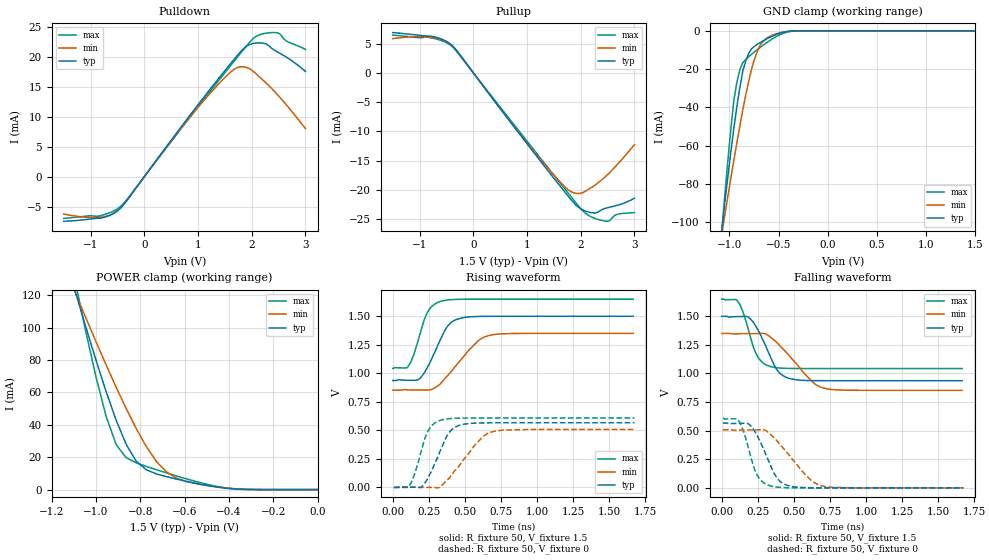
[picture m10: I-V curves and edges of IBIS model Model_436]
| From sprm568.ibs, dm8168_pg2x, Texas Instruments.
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| Model based on original model for BSHTLTCSCDDVGPBFZ
|   Sub model SLOW_5MA_10PER_N_1P5
[model]   Model_436
|[Description]  [1.5V-3-STATE-X-SLOW:5MA, IND, 10%]
|   Slow slew rate (SR[1:0] = "01"), 1.60 * RExt = 0.625 * Iout
|   (I[2:0] = "000"), 5mA nominal with Rext = 50R, ,Industrial
|   temperature range (-40C to 125C, 25C nominal),10% power supply
|   tolerance
|[Input Load]
|[Output Drive] SLOW:5MA
|Voltage   1.5V
|Mode   3-STATE
Model_type   3-state
Polarity   Non-Inverting
Enable   Active-Low
Cref =  15.0000pF
Rref =  100.0000M
Vref =  0V
Vmeas =  0.75
C_comp   1.5249p   1.4275p   1.6205p
[Model Spec]
[Temperature Range]   25   125   -40
[Voltage Range]   1.5   1.35   1.65
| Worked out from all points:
|   slope of the pulldown table from 0 to 0.225 V, typ, clamps not added: 81.7 ohm
|   slope of the pullup table from 0 to 0.225 V, typ, clamps not added: 81.7 ohm
|   GND clamp passes 1 mA (typ) near -0.47 V on its own axis
|   POWER clamp passes 1 mA (typ) near -0.42 V on its own axis
|   rising waveform, R_fixture 50, V_fixture 1.5: 20-80 % time 127ps typ, 205ps min, 93.4ps max; typ from 0.937 V to 1.5 V
|   rising waveform, R_fixture 50, V_fixture 0: 20-80 % time 121ps typ, 192ps min, 89ps max; typ from 0 V to 0.566 V
|   falling waveform, R_fixture 50, V_fixture 1.5: 20-80 % time 126ps typ, 213ps min, 92.7ps max; typ from 1.5 V to 0.937 V
|   falling waveform, R_fixture 50, V_fixture 0: 20-80 % time 122ps typ, 205ps min, 89.1ps max; typ from 0.566 V to 0 V
[POWER_clamp]
-1.5V     321.6mA    260.6mA    415.8mA
-1.091V   121.1mA    120.8mA    126.6mA
-1.076V   114.1mA    115.8mA    116.8mA
-1V       79.88mA    91.3mA     69.56mA
-954.5mV  60.58mA    77.05mA    45.34mA
-909.1mV  42.84mA    63.2mA     27.8mA
-818.2mV  17.47mA    37.6mA     16.51mA
-772.7mV  12.19mA    26.53mA    14.33mA
-681.8mV  7.985mA    10.89mA    10.33mA
-590.9mV  5.092mA    4.952mA    6.596mA
-363.6mV  298.9uA    465.6uA    298.1uA
0V        1.518nA    23.05nA    396.5pA
[Pulldown]
-1.5V     -7.45mA    -6.24mA    -6.96mA
-863.6mV  -6.95mA    -6.794mA   -6.6mA
-500mV    -5.682mA   -5.687mA   -5.359mA
-318.2mV  -3.897mA   -3.877mA   -3.74mA
1V        12mA       11.57mA    11.65mA
1.455V    17.18mA    16.12mA    16.83mA
1.727V    20.16mA    18.19mA    19.88mA
2V        22.16mA    17.76mA    22.81mA
2.318V    21.82mA    15.17mA    23.99mA
2.5V      20.69mA    13.46mA    23.94mA
2.636V    19.99mA    12.06mA    22.66mA
3V        17.55mA    8mA        21.21mA
[Pullup]
-1.5V     6.87mA     5.84mA     6.44mA
-818.2mV  6.271mA    6.054mA    6.043mA
-409.1mV  4.8mA      4.74mA     4.606mA
1.227V    -14.81mA   -14.54mA   -14.31mA
1.682V    -20.1mA    -19.29mA   -19.58mA
1.864V    -22.13mA   -20.48mA   -21.67mA
2V        -23.22mA   -20.59mA   -23.2mA
2.182V    -23.86mA   -19.71mA   -24.55mA
2.409V    -23.31mA   -18.15mA   -25.25mA
2.545V    -22.95mA   -16.97mA   -25.21mA
2.682V    -22.64mA   -15.67mA   -24.17mA
3V        -21.43mA   -12.28mA   -23.87mA
[GND_clamp]
-1.5V     -310mA     -250.5mA   -402.4mA
-1.076V   -103.5mA   -106.1mA   -105.2mA
-1.045V   -89.74mA   -96.32mA   -85.93mA
-954.5mV  -51.19mA   -67.85mA   -36.85mA
-924.2mV  -40.06mA   -58.84mA   -27.27mA
-863.6mV  -21.23mA   -41.55mA   -16.73mA
-833.3mV  -15.79mA   -33.74mA   -15.03mA
-772.7mV  -9.342mA   -19.74mA   -12.19mA
-712.1mV  -6.927mA   -10.35mA   -9.702mA
-621.2mV  -4.26mA    -3.894mA   -6.224mA
-409.1mV  -336.9uA   -288.9uA   -618.6uA
1.5V      1.518nA    2.298uA    269.6pA
[Ramp]
dV/dt_f   0.450816/0.19018024n   0.398752/0.29974943n   0.486/0.1457648n
dV/dt_r  0.4545976/0.18117279n 0.40958896/0.27476076n 0.48679282/0.14067755n
R_load = 50
[Rising Waveform]
R_fixture = 50
V_fixture = 1.5
V_fixture_min = 1.35
V_fixture_max = 1.65
0s        937.3mV    852.6mV    1.043V
105.1ps   939.6mV    855.1mV    1.057V
188ps     954.9mV    853.6mV    1.341V
246.5ps   1.067V     853.5mV    1.546V
337.4ps   1.314V     918.2mV    1.632V
385.5ps   1.421V     986.7mV    1.643V
441.2ps   1.472V     1.072V     1.648V
591.5ps   1.498V     1.284V     1.65V
666.2ps   1.5V       1.331V     1.65V
1.667ns   1.5V       1.35V      1.65V
[Rising Waveform]
R_fixture = 50
V_fixture = 0
V_fixture_min = 0
V_fixture_max = 0
8.2ps     0V         0V         0V
111.8ps   3.026mV    2.887mV    9.648mV
152.4ps   2.107mV    2.335mV    119.8mV
199.5ps   5.554mV    0V         326.1mV
251.8ps   103.7mV    0V         509.5mV
344.9ps   364.6mV    22.9mV     593.6mV
434.2ps   528.9mV    151.8mV    605.9mV
566.8ps   563.2mV    366.6mV    608.2mV
674.1ps   565.9mV    481.5mV    608.4mV
1.675ns   566.4mV    508.1mV    608.4mV
[Falling Waveform]
R_fixture = 50
V_fixture = 1.5
V_fixture_min = 1.35
V_fixture_max = 1.65
0s        1.499V     1.349V     1.649V
108.6ps   1.497V     1.346V     1.635V
189.9ps   1.487V     1.349V     1.361V
249.3ps   1.385V     1.349V     1.147V
342.5ps   1.133V     1.312V     1.058V
393.9ps   1.015V     1.255V     1.048V
449.5ps   963.9mV    1.182V     1.044V
631.7ps   937.3mV    923.7mV    1.042V
722.7ps   936.7mV    867.1mV    1.042V
1.667ns   936.6mV    851.7mV    1.042V
[Falling Waveform]
R_fixture = 50
V_fixture = 0
V_fixture_min = 0
V_fixture_max = 0
8.2ps     565.8mV    507.3mV    607.8mV
117.7ps   563mV      504.8mV    586.7mV
196.9ps   547.4mV    506.7mV    293.9mV
251.5ps   444mV      507.2mV    99.92mV
327.4ps   228.5mV    480mV      21.63mV
374.8ps   102.7mV    422.6mV    7.977mV
423ps     40.2mV     351.5mV    3.196mV
611.4ps   0V         75.93mV    0V
690.9ps   0V         18.69mV    0V
1.675ns   0V         0V         0V
